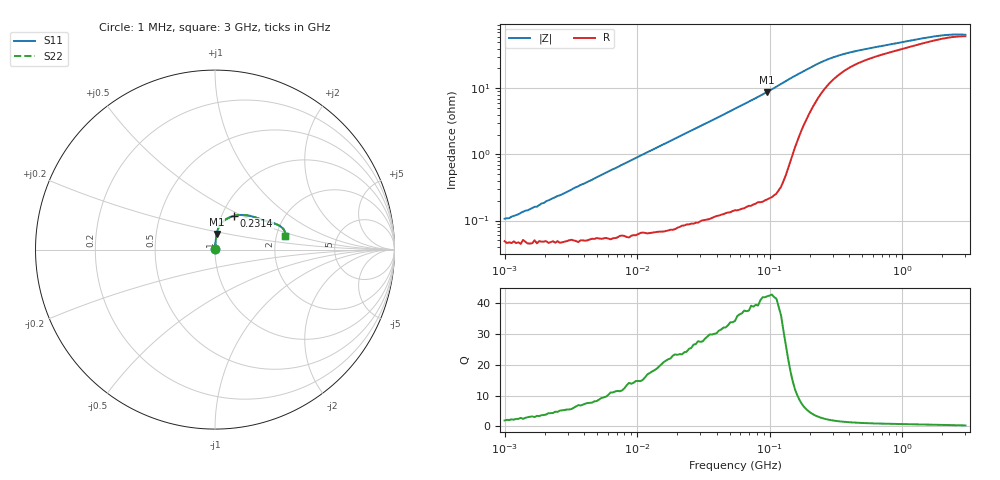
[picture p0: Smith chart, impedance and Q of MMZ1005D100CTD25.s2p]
! S-Parameter Data Generated by TDK Corporation
! Copyright(C) 2025 TDK Corporation.
! All Rights Reserved.
! TDK P/N: MMZ1005D100CTD25 (Chip Bead)
! Property: |Z|=10ohm at 100MHz
! Size(LxWxT): 1x0.5x0.5mm
! Model Type: s2p (Touchstone File Format Version 1.0)
! Frequency: DC=Yes Start=1MHz Stop=3000MHz 202points Log-sweep
! Model Generated on Feb. 6, 2025
! Terms and conditions regarding TDK Simulation Models:
! 1)This simulation model is being provided solely for informational
!  purposes. Please refer to the specifications of the products in
!  terms of detailed characteristics of such products.
! 2)In no event shall TDK Corporation of any of its subsidiaries be
!  liable for any loss or damage arising, directly or indirectly,
!  from any information contained in this simulation model, including,
!  but not limited to loss or damages arising from any inaccuracies,
!  omissions or errors in connection with such information.
! 3)Any and all copyrights on this simulation model are owned by
!  TDK Corporation.  Duplication or redistribution of this simulation
!  model without prior written permission from TDK Corporation
!  is prohibited.
! 4)This simulation model is subject to any modification or change
!  without any prior notice.
! 5)Neither TDK Corporation nor any of its subsidiaries shall make any
!  warranty, express or implied, including but not limited to the
!  correctness, implied warranties of merchantability and fitness for
!  a particular purpose with respect to this simulation models.
! 6)The use of this simulation model shall be deemed to have consented
!  to the terms and conditions hereof.
! Port Assignments:
!  1 ---@@@--- 2
! Applicable Conditions:
!  Temperature = 25 degC
!  DC Bias Current = 0 A
!  Small Signal Operation
# Hz S MA R 50
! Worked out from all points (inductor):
!   201 points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, 1 MHz to 3 GHz, reference 50 ohm
!   read as one part in series: L = 14.5 nH near 1.492 MHz
!   highest Q = 42.2 at 95.93 MHz (marker M1), where L = 14.7 nH
!   S11 on the Smith chart (normalised r, x): 1 MHz: 1.00, +0.00; 231.4 MHz: 1.14, +0.45; 3 GHz: 2.23, +0.40
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1000000  0.001065 62.7  0.9995 -0.1  0.9995 -0.1  0.001065 62.7
1083356  0.001087 64.4  0.9995 -0.1  0.9995 -0.1  0.001087 64.4
1127605  0.001145 66.4  0.9995 -0.1  0.9995 -0.1  0.001145 66.4
1271492  0.001244 67.8  0.9995 -0.1  0.9995 -0.1  0.001244 67.8
1682724  0.001613 71.7  0.9995 -0.1  0.9995 -0.1  0.001613 71.7
1751453  0.001623 73.7  0.9995 -0.1  0.9995 -0.1  0.001623 73.7
1897447  0.001813 74.6  0.9995 -0.1  0.9995 -0.1  0.001813 74.6
1974946  0.001847 74.8  0.9995 -0.1  0.9995 -0.1  0.001847 74.8
2055611  0.001956 75.4  0.9995 -0.1  0.9995 -0.1  0.001956 75.4
2613693  0.002408 78.8  0.9995 -0.1  0.9995 -0.1  0.002408 78.8
3900413  0.003577 81.7  0.9995 -0.2  0.9995 -0.2  0.003577 81.7
1.461624e7  0.01316 86.3  0.9992 -0.8  0.9992 -0.8  0.01316 86.3
5.477226e7  0.04894 85.5  0.9974 -2.8  0.9974 -2.8  0.04894 85.5
9.593103e7  0.08785 83.6  0.9941 -5.0  0.9941 -5.0  0.08785 83.6
1.49005e8  0.1447 77.8  0.9798 -8.3  0.9798 -8.3  0.1447 77.8
2.136344e8  0.2024 64.3  0.9302 -11.3  0.9302 -11.3  0.2024 64.3
2.314421e8  0.2157 60.7  0.9139 -11.9  0.9139 -11.9  0.2157 60.7
2.827291e8  0.2448 52.1  0.8713 -12.8  0.8713 -12.8  0.2448 52.1
3.594878e8  0.2714 43.7  0.8255 -13.1  0.8255 -13.1  0.2714 43.7
8.005644e8  0.3324 28.1  0.724 -12.5  0.724 -12.5  0.3324 28.1
1.855641e9  0.3947 17.8  0.6357 -10.9  0.6357 -10.9  0.3947 17.8
3e9  0.3974 11.1  0.6148 -7.1  0.6148 -7.1  0.3974 11.1
